(* Logix 5000 Program export KEP; software revision 30.00 *)

TYPE EdDSA_INTERNAL :
STRUCT
   MsgCopy : EdDSA_MSG;
   MsgToBeVerified : EdDSA_MSG;
   MsgLastVerified : EdDSA_MSG;
   MsgInProcessing : EdDSA_MSG;
   MsgToBeSent : EdDSA_MSG;
   VerifyQue : DINT;
   ProcessQue : DINT;
   VerificationInProgress : BOOL;
   VerificationStatus : DINT;
   ProcessingRequired : BOOL;
   ProcessingInProgress : BOOL;
   ProcessingStatus : DINT;
END_STRUCT
END_TYPE

TYPE EdDSA_MSG :
STRUCT
   Status : CONNECTION_STATUS;
   Flags : DINT;
   PubDH : STRING;
   Ke : STRING;
   KsID : LINT;
   KsPrimeID : LINT;
   Counter : LINT;
   Sig_R : STRING;
   Sig_S : STRING;
END_STRUCT
END_TYPE

TYPE EdDSA_STATECTRL :
STRUCT
   RESET : BOOL;
   DN : BOOL;
   START : BOOL;
   ONS : INT;
   STEP : INT;
   CMD : INT;
   CMD_TABLE : INT[20];
   DONE : INT;
   NEXT_STEP : INT;
   TIMER : TIMER[5];
   NEXT_STATE : INT;
   TEMP : DINT[5];
END_STRUCT
END_TYPE

TYPE InternalFlags :
STRUCT
   KsPrimeRequest : BOOL;
   CreateNewKsPrimeRequest : BOOL;
   KsIDMatchesMe : BOOL;
   KsPrimeIDMatchesMe : BOOL;
   MyPriDH : STRING;
   MyPubDH : STRING;
   PartnerLastPubDH : STRING;
   Ke : STRING;
END_STRUCT
END_TYPE

TYPE POINT :   // A point on an Edwards-curve represented in extended homogeneous coordinates
STRUCT
   X : DINT[22];
   Y : DINT[22];
   Z : DINT[22];
   T : DINT[22];
END_STRUCT
END_TYPE

TYPE Std_DiscreteAlarm :   // ALARM RESET
STRUCT
   AckC : BOOL;   // ALARM ACKNOWLEDGE
   LatchA : BOOL;   // ALARM LATCH
   DetectS : BOOL;   // ALARM DETECT
   BitS : BOOL;   // ALARM MISCOMPARE
   InhibitC : BOOL;   // ALARM INHIBIT
   Tmr : TIMER;   // ALARM Timer
END_STRUCT
END_TYPE

TYPE VMAC_DATA_INTERNAL :
STRUCT
   VMACOK : BOOL;
   CommsOK : BOOL;
   KeyOK : BOOL;
   KsInUse : BOOL;
   KsPrimeInUse : BOOL;
   EntryStatus : INT;
   NodeID : DINT;
   DestinationID : DINT;
   Counter : LINT;
   LastCounter : LINT;
   KeyID : LINT;
   VMAC_KEY : DINT[8];
   VMAC_CALC : DINT[8];
   VMAC_INPUT : DINT[8];
   DATA_INPUT : DINT[1600];
   DATA_VERIFIED : DINT[1600];
   VMAC_CTRL : VMAC;
   KeyAlarm : Std_DiscreteAlarm;
   ReplayAlarm : Std_DiscreteAlarm;
   InvalidAlarm : Std_DiscreteAlarm;
   NodeAlarm : Std_DiscreteAlarm;
   DestinationAlarm : Std_DiscreteAlarm;
   L_LES : L_LES;
   L_EQU : L_EQU;
   CommsTimer : TIMER;
END_STRUCT
END_TYPE

ADD_ON_INSTRUCTION B256_ADD   (* revision 1.0 20170916, vendor Kenneth A. Fischer *)
// c3=c1+c2 with no reduction
// Revision note:
// Rev1.0: 20170916 - Initial Release
VAR_IN_OUT
   Inp_C1 : DINT[22]; {required}
   Inp_C2 : DINT[22]; {required}
   Out_C3 : DINT[22]; {required}
END_VAR
VAR
   i : INT;
END_VAR

ROUTINE Logic   (* ladder *)
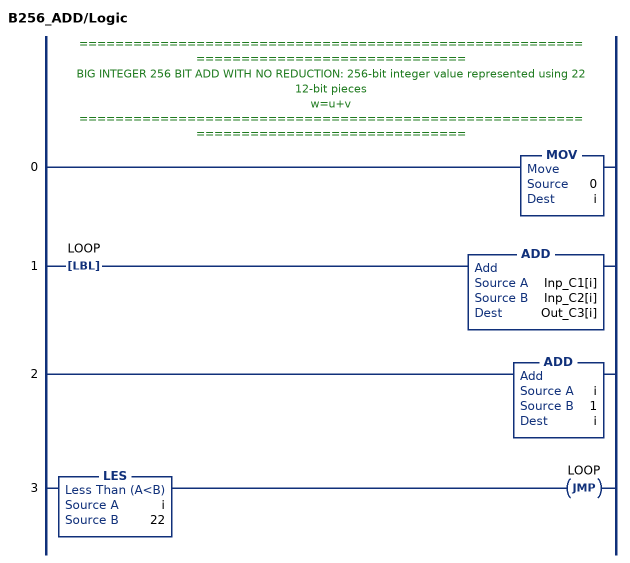
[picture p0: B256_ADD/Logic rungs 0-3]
   // ======================================================================================
   // BIG INTEGER 256 BIT ADD WITH NO REDUCTION: 256-bit integer value represented using 22 12-bit pieces
   // w=u+v
   // ======================================================================================
   0: MOV(0,i);
   1: LBL(LOOP)ADD(Inp_C1[i],Inp_C2[i],Out_C3[i]);
   2: ADD(i,1,i);
   3: LES(i,22)JMP(LOOP);
END_ROUTINE
END_ADD_ON_INSTRUCTION

ADD_ON_INSTRUCTION D_SHR   (* revision 1.0 20170524, vendor Kenneth A. Fischer *)
// DINT bit shift right of the 32-bit argument Inp_A by Inp_B bits with paddding by zeros on the right
// Revision note:
// Rev1.0: 20170524 - Initial Release
VAR_IN_OUT
   Inp_A : DINT; {required}   // 64-bit Integer to be right circular rotated
END_VAR
VAR_INPUT
   Inp_B : INT; {required}   // Number of bits to shift
END_VAR
VAR_IN_OUT
   Out : DINT; {required}   // Result
END_VAR
VAR
   BSR_Cntrl : CONTROL := (LEN := 32);
   ONS : BOOL;
   Source_Bit : BOOL;
   Wrk_InpA : DINT[2];
END_VAR

ROUTINE Logic   (* ladder *)
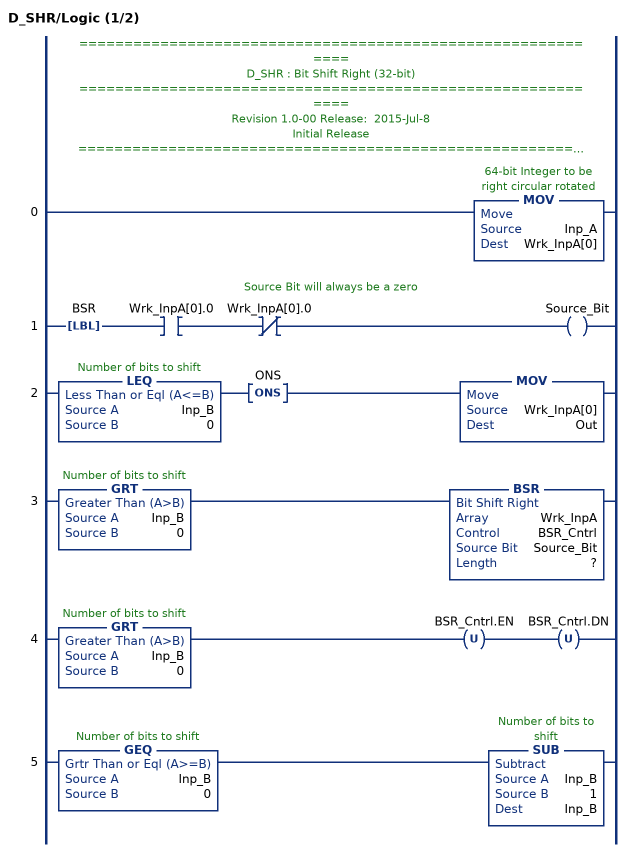
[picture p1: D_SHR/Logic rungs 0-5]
   // ============================================================
   // D_SHR : Bit Shift Right (32-bit)
   // ============================================================
   // Revision 1.0-00 Release:  2015-Jul-8
   // Initial Release
   // ============================================================
   // Performs a right bit shift of the 32-bit argument Inp_A by the
   // number of bits defined in the 16-bit argument Inp_B, with padding by zeros.
   0: MOV(Inp_A,Wrk_InpA[0]);
   // Source Bit will always be a zero
   1: LBL(BSR)XIC(Wrk_InpA[0].0)XIO(Wrk_InpA[0].0)OTE(Source_Bit);
   2: LEQ(Inp_B,0)ONS(ONS)MOV(Wrk_InpA[0],Out);
   3: GRT(Inp_B,0)BSR(Wrk_InpA,BSR_Cntrl,Source_Bit,?);
   4: GRT(Inp_B,0)OTU(BSR_Cntrl.EN)OTU(BSR_Cntrl.DN);
   5: GEQ(Inp_B,0)SUB(Inp_B,1,Inp_B);
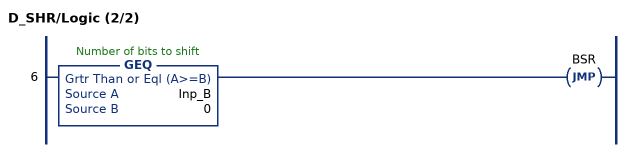
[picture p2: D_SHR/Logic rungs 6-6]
   6: GEQ(Inp_B,0)JMP(BSR);
END_ROUTINE
END_ADD_ON_INSTRUCTION

ADD_ON_INSTRUCTION B256_NRED   (* revision 1.0 20170916, vendor Kenneth A. Fischer *)
// Reduce 256-bit integer stored in 22 pieces by propagating carries
// Revision note:
// Rev1.0: 20170916 - Initial Release
VAR_IN_OUT
   Inp_C : DINT[22]; {required}
END_VAR
VAR
   D_SHR : D_SHR;
   temp : DINT;
   i : INT;
END_VAR

ROUTINE Logic   (* ladder *)
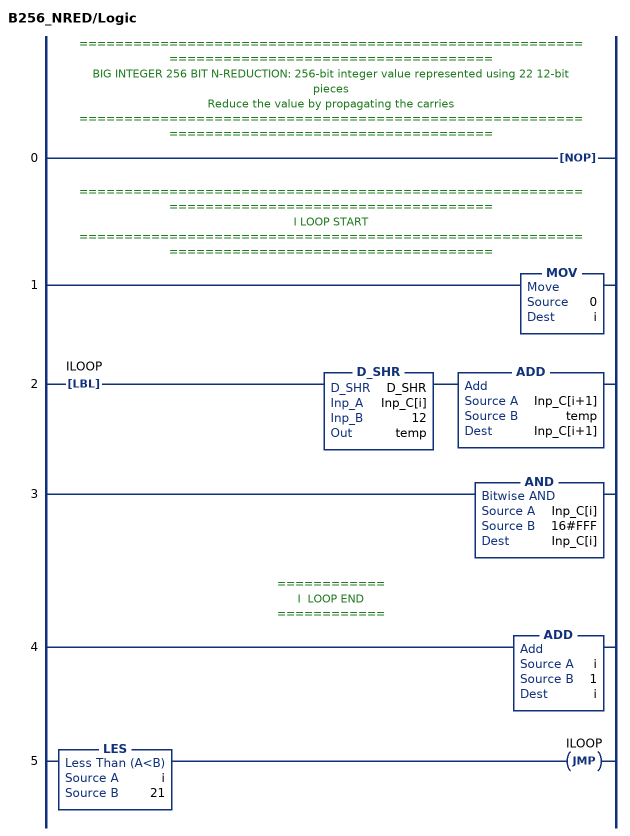
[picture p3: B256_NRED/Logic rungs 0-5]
   // ============================================================================================
   // BIG INTEGER 256 BIT N-REDUCTION: 256-bit integer value represented using 22 12-bit pieces
   // Reduce the value by propagating the carries
   // ============================================================================================
   0: NOP();
   // ============================================================================================
   // I LOOP START
   // ============================================================================================
   1: MOV(0,i);
   2: LBL(ILOOP)D_SHR(D_SHR,Inp_C[i],12,temp)ADD(Inp_C[i+1],temp,Inp_C[i+1]);
   3: AND(Inp_C[i],16#FFF,Inp_C[i]);
   // ============
   // I  LOOP END
   // ============
   4: ADD(i,1,i);
   5: LES(i,21)JMP(ILOOP);
END_ROUTINE
END_ADD_ON_INSTRUCTION

ADD_ON_INSTRUCTION B256_SUB   (* revision 1.0 20170916, vendor Kenneth A. Fischer *)
// c3=c1-c2 with reduction
// Revision note:
// Rev1.0: 20170916 - Initial Release
VAR_IN_OUT
   Inp_C1 : DINT[22]; {required}
   Inp_C2 : DINT[22]; {required}
   Out_C3 : DINT[22]; {required}
END_VAR
VAR
   B256_ADD : B256_ADD;
   B256_NRED : B256_NRED;
   temp : DINT;
   i : INT;
END_VAR

ROUTINE Logic   (* ladder *)
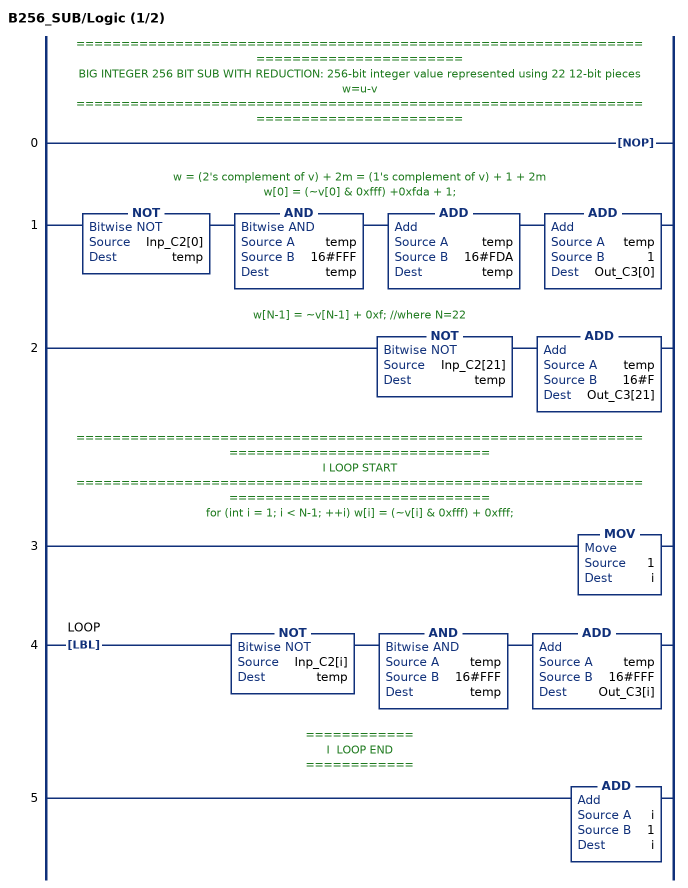
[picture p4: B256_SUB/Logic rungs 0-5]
   // ======================================================================================
   // BIG INTEGER 256 BIT SUB WITH REDUCTION: 256-bit integer value represented using 22 12-bit pieces
   //  w=u-v
   // ======================================================================================
   0: NOP();
   // w = (2's complement of v) + 2m = (1's complement of v) + 1 + 2m
   // w[0] = (~v[0] & 0xfff) +0xfda + 1;
   1: NOT(Inp_C2[0],temp)AND(temp,16#FFF,temp)ADD(temp,16#FDA,temp)ADD(temp,1,Out_C3[0]);
   // w[N-1] = ~v[N-1] + 0xf; //where N=22
   2: NOT(Inp_C2[21],temp)ADD(temp,16#F,Out_C3[21]);
   // ============================================================================================
   // I LOOP START
   // ============================================================================================
   // for (int i = 1; i < N-1; ++i) w[i] = (~v[i] & 0xfff) + 0xfff;
   3: MOV(1,i);
   4: LBL(LOOP)NOT(Inp_C2[i],temp)AND(temp,16#FFF,temp)ADD(temp,16#FFF,Out_C3[i]);
   // ============
   // I  LOOP END
   // ============
   5: ADD(i,1,i);
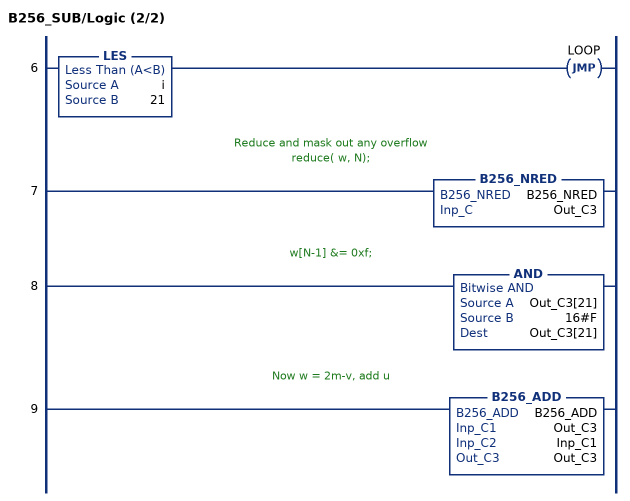
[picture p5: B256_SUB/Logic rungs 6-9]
   6: LES(i,21)JMP(LOOP);
   // Reduce and mask out any overflow
   // reduce( w, N);
   7: B256_NRED(B256_NRED,Out_C3);
   // w[N-1] &= 0xf;
   8: AND(Out_C3[21],16#F,Out_C3[21]);
   // Now w = 2m-v, add u
   9: B256_ADD(B256_ADD,Out_C3,Inp_C1,Out_C3);
END_ROUTINE
END_ADD_ON_INSTRUCTION

ADD_ON_INSTRUCTION B256_FRED   (* revision 1.0 20170916, vendor Kenneth A. Fischer *)
// fast_reduce:  reduce by propagating the carries starting at a particular offset and stoping once the carry becomes zero
// Revision note:
// Rev1.0: 20170916 - Initial Release
VAR_IN_OUT
   Inp_C : DINT[22]; {required}
END_VAR
VAR_INPUT
   Inp_offset : INT; {required}
END_VAR
VAR
   i : INT;
   carry : DINT;
   D_SHR : D_SHR;
END_VAR

ROUTINE Logic   (* ladder *)
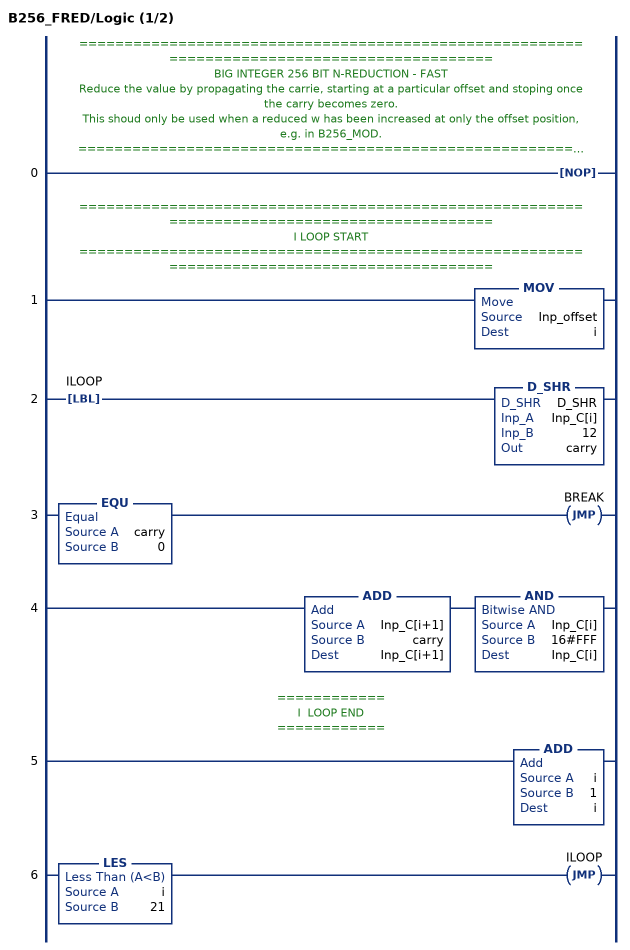
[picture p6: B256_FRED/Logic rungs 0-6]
   // ============================================================================================
   // BIG INTEGER 256 BIT N-REDUCTION - FAST
   // Reduce the value by propagating the carrie, starting at a particular offset and stoping once the carry becomes zero.
   // This shoud only be used when a reduced w has been increased at only the offset position, e.g. in B256_MOD.
   // ============================================================================================
   0: NOP();
   // ============================================================================================
   // I LOOP START
   // ============================================================================================
   1: MOV(Inp_offset,i);
   2: LBL(ILOOP)D_SHR(D_SHR,Inp_C[i],12,carry);
   3: EQU(carry,0)JMP(BREAK);
   4: ADD(Inp_C[i+1],carry,Inp_C[i+1])AND(Inp_C[i],16#FFF,Inp_C[i]);
   // ============
   // I  LOOP END
   // ============
   5: ADD(i,1,i);
   6: LES(i,21)JMP(ILOOP);
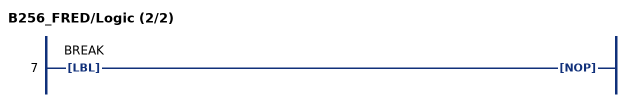
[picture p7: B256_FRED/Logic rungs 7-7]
   7: LBL(BREAK)NOP();
END_ROUTINE
END_ADD_ON_INSTRUCTION

ADD_ON_INSTRUCTION D_SHL   (* revision 1.0 20170524, vendor Kenneth A. Fischer *)
// DINT bit shift left of the 32-bit argument Inp_A by Inp_B bits with paddding by zeros on the right
// Revision note:
// Rev1.0: 20170524 - Initial Release
VAR_IN_OUT
   Inp_A : DINT; {required}   // 64-bit Integer to be right circular rotated
END_VAR
VAR_INPUT
   Inp_B : INT; {required}   // Number of bits to shift
END_VAR
VAR_IN_OUT
   Out : DINT; {required}   // Result
END_VAR
VAR
   Wrk_InpA : DINT[2];
   Source_Bit : BOOL;
   ONS : BOOL;
   BSL_Cntrl : CONTROL := (LEN := 32);
END_VAR

ROUTINE Logic   (* ladder *)
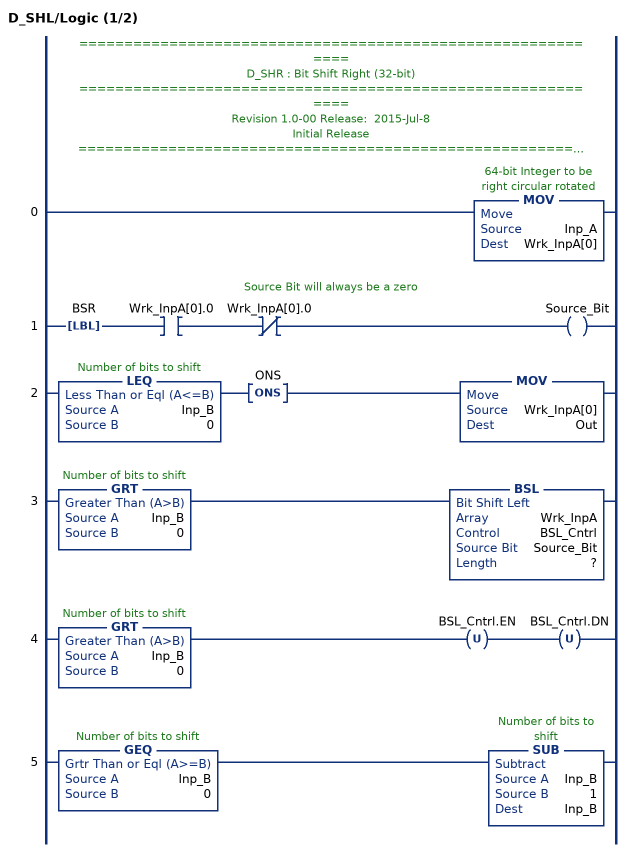
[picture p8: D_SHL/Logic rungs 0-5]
   // ============================================================
   // D_SHR : Bit Shift Right (32-bit)
   // ============================================================
   // Revision 1.0-00 Release:  2015-Jul-8
   // Initial Release
   // ============================================================
   // Performs a left bit shift of the 32-bit argument Inp_A by the
   // number of bits defined in the 16-bit argument Inp_B, with padding by zeros.
   0: MOV(Inp_A,Wrk_InpA[0]);
   // Source Bit will always be a zero
   1: LBL(BSR)XIC(Wrk_InpA[0].0)XIO(Wrk_InpA[0].0)OTE(Source_Bit);
   2: LEQ(Inp_B,0)ONS(ONS)MOV(Wrk_InpA[0],Out);
   3: GRT(Inp_B,0)BSL(Wrk_InpA,BSL_Cntrl,Source_Bit,?);
   4: GRT(Inp_B,0)OTU(BSL_Cntrl.EN)OTU(BSL_Cntrl.DN);
   5: GEQ(Inp_B,0)SUB(Inp_B,1,Inp_B);
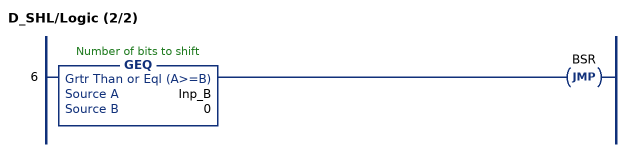
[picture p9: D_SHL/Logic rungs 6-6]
   6: GEQ(Inp_B,0)JMP(BSR);
END_ROUTINE
END_ADD_ON_INSTRUCTION

ADD_ON_INSTRUCTION B256_MOD   (* revision 1.0 20170916, vendor Kenneth A. Fischer *)
// c = d mod (2^255 - 19)
// Revision note:
// Rev1.0: 20170916 - Initial Release
VAR_IN_OUT
   Inp_D : DINT[43]; {required}
   Out_C : DINT[22]; {required}
END_VAR
VAR
   B256_NRED : B256_NRED;
   D_SHL : D_SHL;
   D_SHR : D_SHR;
   i : INT;
   t : DINT;
   temp : DINT;
   temp2 : DINT;
   B256_FRED : B256_FRED;
   offset : DINT;
END_VAR

ROUTINE Logic   (* ladder *)
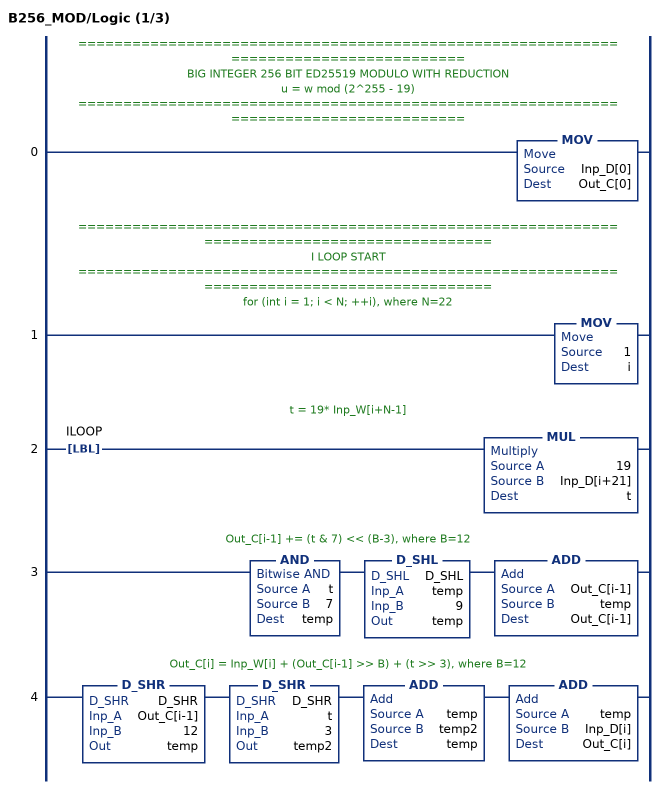
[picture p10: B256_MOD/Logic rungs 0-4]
   // ======================================================================================
   // BIG INTEGER 256 BIT ED25519 MODULO WITH REDUCTION
   //  u = w mod (2^255 - 19)
   // ======================================================================================
   0: MOV(Inp_D[0],Out_C[0]);
   // ============================================================================================
   // I LOOP START
   // ============================================================================================
   // for (int i = 1; i < N; ++i), where N=22
   1: MOV(1,i);
   // t = 19* Inp_W[i+N-1]
   2: LBL(ILOOP)MUL(19,Inp_D[i+21],t);
   // Out_C[i-1] += (t & 7) << (B-3), where B=12
   3: AND(t,7,temp)D_SHL(D_SHL,temp,9,temp)ADD(Out_C[i-1],temp,Out_C[i-1]);
   // Out_C[i] = Inp_W[i] + (Out_C[i-1] >> B) + (t >> 3), where B=12
   4: D_SHR(D_SHR,Out_C[i-1],12,temp)D_SHR(D_SHR,t,3,temp2)ADD(temp,temp2,temp)ADD(temp,Inp_D[i],Out_C[i]);
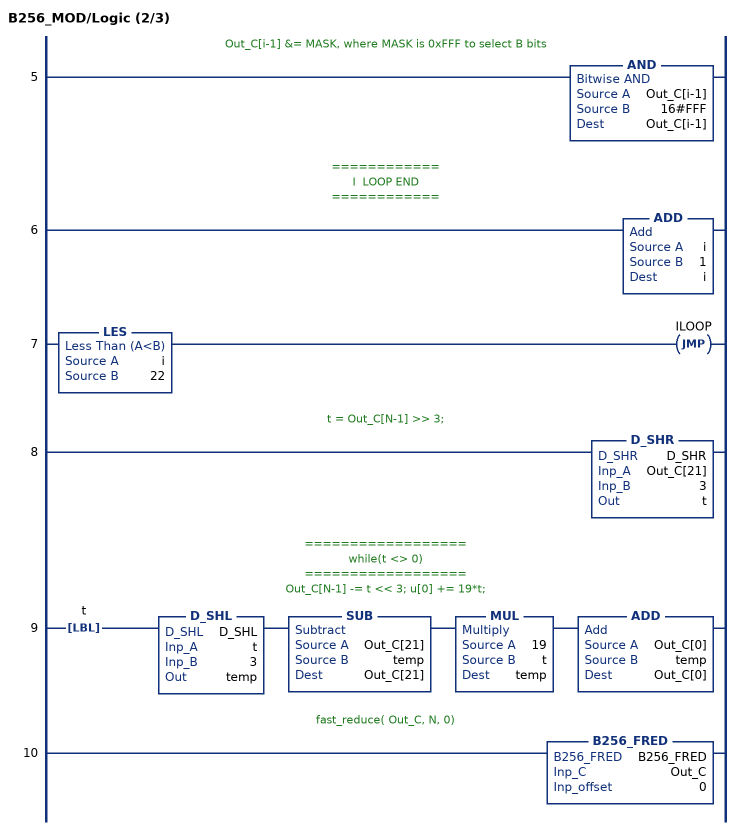
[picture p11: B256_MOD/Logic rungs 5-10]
   // Out_C[i-1] &= MASK, where MASK is 0xFFF to select B bits
   5: AND(Out_C[i-1],16#FFF,Out_C[i-1]);
   // ============
   // I  LOOP END
   // ============
   6: ADD(i,1,i);
   7: LES(i,22)JMP(ILOOP);
   // t = Out_C[N-1] >> 3;
   8: D_SHR(D_SHR,Out_C[21],3,t);
   // ==================
   // while(t <> 0)
   // ==================
   // Out_C[N-1] -= t << 3; u[0] += 19*t;
   9: LBL(t)D_SHL(D_SHL,t,3,temp)SUB(Out_C[21],temp,Out_C[21])MUL(19,t,temp)ADD(Out_C[0],temp,Out_C[0]);
   // fast_reduce( Out_C, N, 0)
   10: B256_FRED(B256_FRED,Out_C,0);
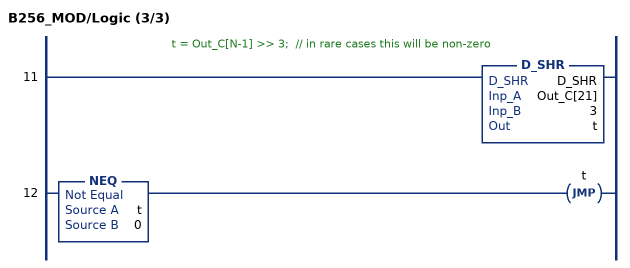
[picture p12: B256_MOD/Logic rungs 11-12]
   // t = Out_C[N-1] >> 3;  // in rare cases this will be non-zero
   11: D_SHR(D_SHR,Out_C[21],3,t);
   12: NEQ(t,0)JMP(t);
END_ROUTINE
END_ADD_ON_INSTRUCTION

ADD_ON_INSTRUCTION B256_NNRED   (* revision 1.0 20170916, vendor Kenneth A. Fischer *)
// Reduce 256-bit integer stored in 43 pieces by propagating carries
// Revision note:
// Rev1.0: 20170916 - Initial Release
VAR_IN_OUT
   Inp_D : DINT[43]; {required}
END_VAR
VAR
   temp : DINT;
   i : INT;
   D_SHR : D_SHR;
END_VAR

ROUTINE Logic   (* ladder *)
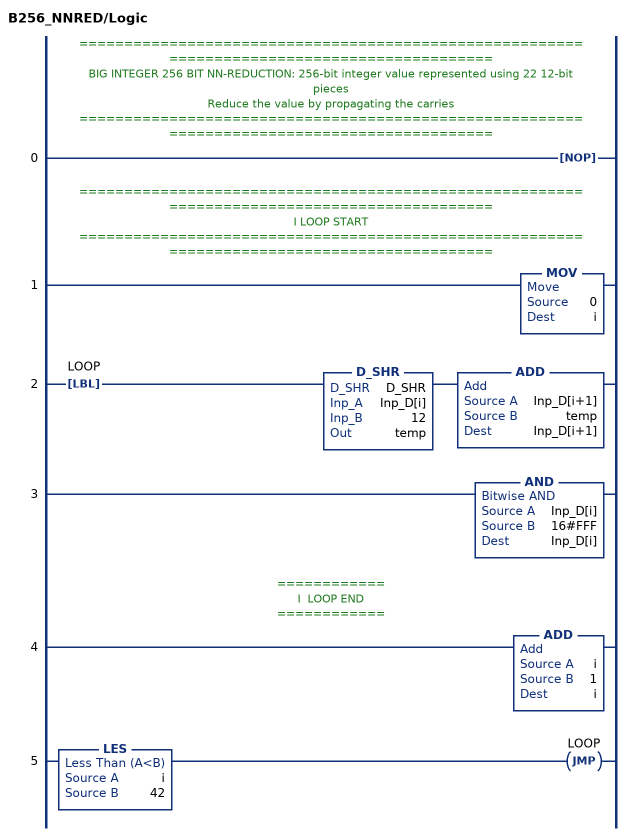
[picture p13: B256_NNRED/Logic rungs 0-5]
   // ============================================================================================
   // BIG INTEGER 256 BIT NN-REDUCTION: 256-bit integer value represented using 22 12-bit pieces
   // Reduce the value by propagating the carries
   // ============================================================================================
   0: NOP();
   // ============================================================================================
   // I LOOP START
   // ============================================================================================
   1: MOV(0,i);
   2: LBL(LOOP)D_SHR(D_SHR,Inp_D[i],12,temp)ADD(Inp_D[i+1],temp,Inp_D[i+1]);
   3: AND(Inp_D[i],16#FFF,Inp_D[i]);
   // ============
   // I  LOOP END
   // ============
   4: ADD(i,1,i);
   5: LES(i,42)JMP(LOOP);
END_ROUTINE
END_ADD_ON_INSTRUCTION

ADD_ON_INSTRUCTION B256_MUL   (* revision 1.0 20170916, vendor Kenneth A. Fischer *)
// c3 = c1*c2 with reduction and mod
// Revision note:
// Rev1.0: 20170916 - Initial Release
VAR_IN_OUT
   Temp_D : DINT[43]; {required}
   Inp_C1 : DINT[22]; {required}
   Inp_C2 : DINT[22]; {required}
   Out_C3 : DINT[22]; {required}
END_VAR
VAR
   B256_MOD : B256_MOD;
   B256_NNRED : B256_NNRED;
   i : INT;
   j : INT;
   mul_temp : DINT;
END_VAR

ROUTINE Logic   (* ladder *)
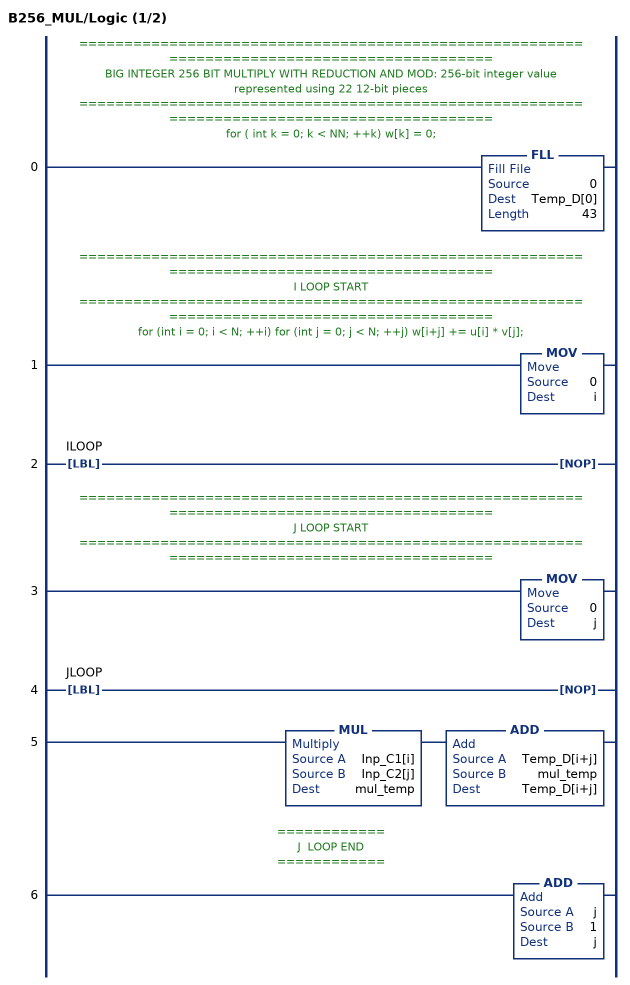
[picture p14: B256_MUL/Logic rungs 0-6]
   // ============================================================================================
   // BIG INTEGER 256 BIT MULTIPLY WITH REDUCTION AND MOD: 256-bit integer value represented using 22 12-bit pieces
   // ============================================================================================
   // for ( int k = 0; k < NN; ++k) w[k] = 0;
   0: FLL(0,Temp_D[0],43);
   // ============================================================================================
   // I LOOP START
   // ============================================================================================
   // for (int i = 0; i < N; ++i) for (int j = 0; j < N; ++j) w[i+j] += u[i] * v[j];
   1: MOV(0,i);
   2: LBL(ILOOP)NOP();
   // ============================================================================================
   // J LOOP START
   // ============================================================================================
   3: MOV(0,j);
   4: LBL(JLOOP)NOP();
   5: MUL(Inp_C1[i],Inp_C2[j],mul_temp)ADD(Temp_D[i+j],mul_temp,Temp_D[i+j]);
   // ============
   // J  LOOP END
   // ============
   6: ADD(j,1,j);
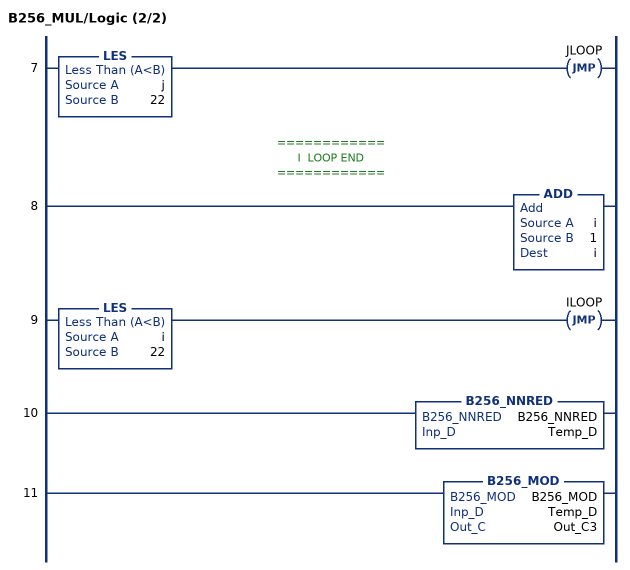
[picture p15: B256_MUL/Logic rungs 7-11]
   7: LES(j,22)JMP(JLOOP);
   // ============
   // I  LOOP END
   // ============
   8: ADD(i,1,i);
   9: LES(i,22)JMP(ILOOP);
   10: B256_NNRED(B256_NNRED,Temp_D);
   11: B256_MOD(B256_MOD,Temp_D,Out_C3);
END_ROUTINE
END_ADD_ON_INSTRUCTION

ADD_ON_INSTRUCTION B256_MUL2   (* revision 1.0 20170916, vendor Kenneth A. Fischer *)
// c3= 2*c1*c2 with reduction and mod
// Revision note:
// Rev1.0: 20170916 - Initial Release
VAR_IN_OUT
   Temp_D : DINT[43]; {required}
   Inp_C1 : DINT[22]; {required}
   Inp_C2 : DINT[22]; {required}
   Out_C3 : DINT[22]; {required}
END_VAR
VAR
   B256_NNRED : B256_NNRED;
   i : INT;
   j : INT;
   mul_temp : DINT;
   B256_MOD : B256_MOD;
   t : DINT;
END_VAR

ROUTINE Logic   (* ladder *)
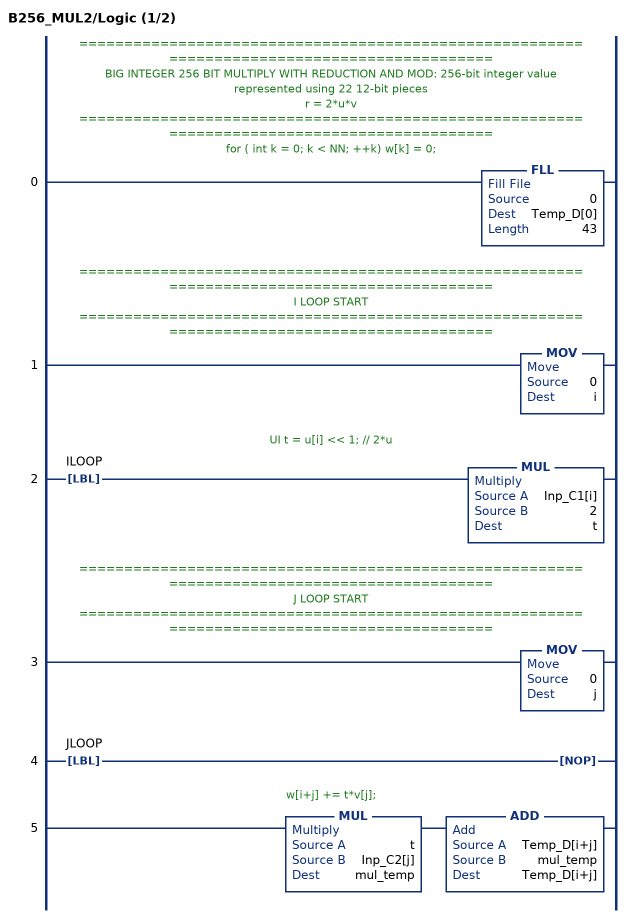
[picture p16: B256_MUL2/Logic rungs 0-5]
   // ============================================================================================
   // BIG INTEGER 256 BIT MULTIPLY WITH REDUCTION AND MOD: 256-bit integer value represented using 22 12-bit pieces
   // r = 2*u*v
   // ============================================================================================
   // for ( int k = 0; k < NN; ++k) w[k] = 0;
   0: FLL(0,Temp_D[0],43);
   // ============================================================================================
   // I LOOP START
   // ============================================================================================
   1: MOV(0,i);
   // UI t = u[i] << 1; // 2*u
   2: LBL(ILOOP)MUL(Inp_C1[i],2,t);
   // ============================================================================================
   // J LOOP START
   // ============================================================================================
   3: MOV(0,j);
   4: LBL(JLOOP)NOP();
   // w[i+j] += t*v[j];
   5: MUL(t,Inp_C2[j],mul_temp)ADD(Temp_D[i+j],mul_temp,Temp_D[i+j]);
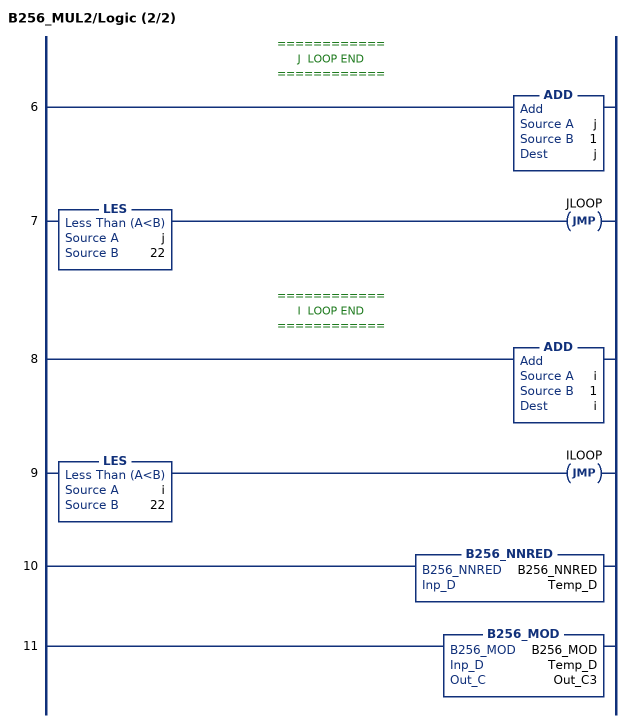
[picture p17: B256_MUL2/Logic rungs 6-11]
   // ============
   // J  LOOP END
   // ============
   6: ADD(j,1,j);
   7: LES(j,22)JMP(JLOOP);
   // ============
   // I  LOOP END
   // ============
   8: ADD(i,1,i);
   9: LES(i,22)JMP(ILOOP);
   10: B256_NNRED(B256_NNRED,Temp_D);
   11: B256_MOD(B256_MOD,Temp_D,Out_C3);
END_ROUTINE
END_ADD_ON_INSTRUCTION
